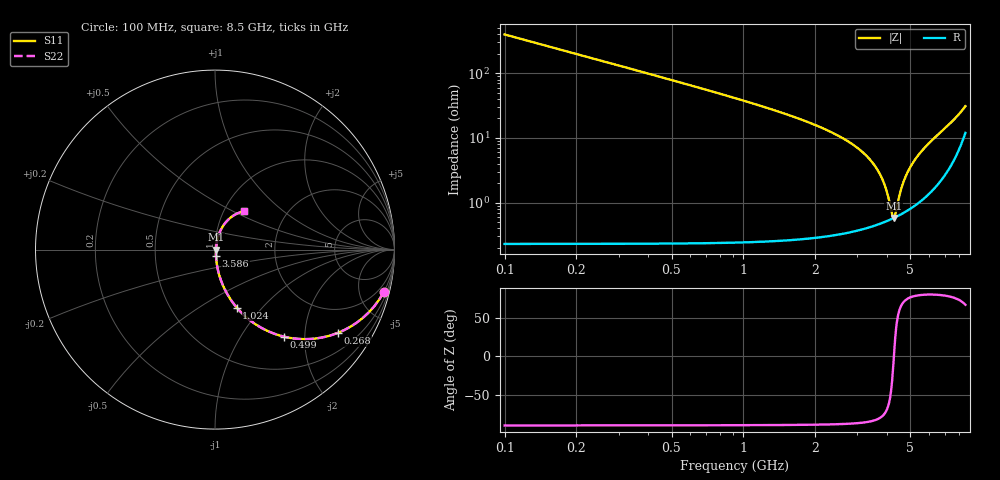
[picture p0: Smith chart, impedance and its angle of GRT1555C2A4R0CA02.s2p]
!Murata Part Number: GRT1555C2A4R0CA02
!These Parameters are Measured in Series Mode Connection
!Data Generated on Jun 19, 2026
!  o--ll--o
!Port1  Port2
!  o------o
!Operation Temp=25[degC], DC Bias Voltage=0[V]
!Freq. Start=100[MHz] Stop=9[GHz] 401[Steps]
# Hz S RI R 50
!Freq.(Hz) S11(Real) S11(Imag) S21(Real) S21(Imag) S12(Real) S12(Imag) S22(Real) S22(Imag)
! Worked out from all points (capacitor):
!   401 points, 100 MHz to 8.5 GHz, reference 50 ohm
!   read as one part in series: C = 4 pF near 142 MHz
!   lowest |Z| = 579 mohm at 4.258 GHz (marker M1)
!   series resonance near 4.265 GHz, so ESL is about 350 pH
!   S11 on the Smith chart (normalised r, x): 100 MHz: 1.00, -7.95; 268 MHz: 1.00, -2.96; 499 MHz: 1.00, -1.57; 1.024 GHz: 1.00, -0.74; 3.586 GHz: 1.01, -0.07; 8.5 GHz: 1.24, +0.57
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1e8  0.9404 -0.2364  0.0596 0.2364  0.0596 0.2364  0.9404 -0.2364
1.84e8  0.8231 -0.3811  0.1769 0.3811  0.1769 0.3811  0.8231 -0.3811
2.68e8  0.6861 -0.4633  0.3139 0.4633  0.3139 0.4633  0.6861 -0.4633
3.73e8  0.5287 -0.4981  0.4713 0.4981  0.4713 0.4981  0.5287 -0.4981
4.99e8  0.3831 -0.4847  0.6169 0.4847  0.6169 0.4847  0.3831 -0.4847
7.3e8  0.2206 -0.4125  0.7794 0.4125  0.7794 0.4125  0.2206 -0.4125
1.024e9  0.121 -0.3228  0.879 0.3228  0.879 0.3228  0.121 -0.3228
1.507e9  0.054 -0.2205  0.946 0.2205  0.946 0.2205  0.054 -0.2205
2.914e9  0.00929 -0.0752  0.9907 0.0752  0.9907 0.0752  0.00929 -0.0752
3.292e9  0.00667 -0.0512  0.9933 0.0512  0.9933 0.0512  0.00667 -0.0512
3.586e9  0.00565 -0.0345  0.9943 0.0345  0.9943 0.0345  0.00565 -0.0345
3.901e9  0.00532 -0.018  0.9947 0.018  0.9947 0.018  0.00532 -0.018
4.027e9  0.00538 -0.0116  0.9946 0.0116  0.9946 0.0116  0.00538 -0.0116
4.195e9  0.00562 -0.00338  0.9944 0.00338  0.9944 0.00338  0.00562 -0.00338
4.258e9  0.00575 -0.000346  0.9943 0.000346  0.9943 0.000346  0.00575 -0.000346
4.3e9  0.00585 0.00167  0.9941 -0.00167  0.9941 -0.00167  0.00585 0.00167
4.552e9  0.00669 0.0135  0.9933 -0.0135  0.9933 -0.0135  0.00669 0.0135
4.804e9  0.00792 0.0251  0.9921 -0.0251  0.9921 -0.0251  0.00792 0.0251
5.182e9  0.0105 0.0423  0.9895 -0.0423  0.9895 -0.0423  0.0105 0.0423
5.707e9  0.0159 0.0663  0.9841 -0.0663  0.9841 -0.0663  0.0159 0.0663
7.114e9  0.0484 0.1371  0.9516 -0.1371  0.9516 -0.1371  0.0484 0.1371
8.5e9  0.1617 0.2142  0.8383 -0.2142  0.8383 -0.2142  0.1617 0.2142
